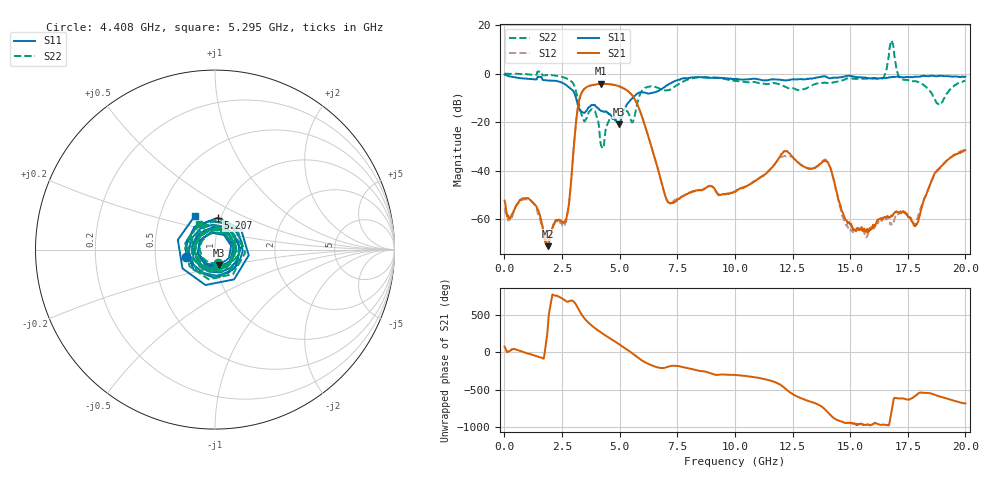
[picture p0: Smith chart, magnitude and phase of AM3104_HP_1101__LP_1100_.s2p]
!Created with skrf (http://scikit-rf.org).
# Hz S RI R 50.0
!freq ReS11 ImS11 ReS21 ImS21 ReS12 ImS12 ReS22 ImS22
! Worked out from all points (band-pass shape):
!   1601 points, 10 MHz to 20 GHz, reference 50 ohm
!   highest |S21| = -4.20 dB at 4.195 GHz (marker M1); lowest = -71.1 dB at 1.872 GHz (marker M2)
!   |S21| within 3 dB of the highest: 3.395 GHz to 5.359 GHz (1.964 GHz wide, 44.9 % of centre)
!   lowest |S11| = -20.9 dB at 4.958 GHz (marker M3), VSWR 1.20, Z = 51.4 - j9.07 ohm
!   |S11| at or under -10 dB: 3.106 GHz to 5.571 GHz (2.465 GHz wide, 56.8 % of centre)
!   |S22| runs from -30.8 to 13.6 dB; largest |S21 - S12| = 0.057
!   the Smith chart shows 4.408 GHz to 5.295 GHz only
!   S11 on the Smith chart (normalised r, x): 4.408 GHz: 0.72, -0.06; 5.207 GHz: 0.97, +0.35; 5.295 GHz: 0.75, +0.30
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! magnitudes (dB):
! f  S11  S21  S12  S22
! 10 MHz  -0.4  -52.3  -55.5  -0.1
! 1.147 GHz  -2.2  -52.3  -52.3  -0.5
! 1.872 GHz  -2.9  -71.1  -67.9  -0.7
! 2.684 GHz  -4.8  -59.9  -60.7  -1.9
! 3.346 GHz  -15.7  -8.0  -8.1  -16.8
! 3.896 GHz  -13.0  -4.6  -4.6  -15.3
! 4.195 GHz  -15.3  -4.2  -4.2  -29.7
! 4.408 GHz  -15.6  -4.3  -4.3  -22.2
! 4.958 GHz  -20.9  -5.2  -5.2  -18.8
! 5.207 GHz  -15.0  -6.3  -6.3  -15.7
! 5.295 GHz  -13.2  -6.8  -6.8  -15.4
! 6.682 GHz  -7.2  -40.0  -40.1  -6.0
! 7.181 GHz  -4.1  -53.3  -53.3  -6.7
! 10.01 GHz  -2.4  -48.7  -48.6  -3.1
! 12.18 GHz  -2.8  -32.0  -34.0  -5.5
! 13.34 GHz  -2.1  -39.2  -39.2  -4.9
! 14.02 GHz  -1.6  -36.4  -36.2  -3.9
! 15.03 GHz  -1.0  -61.9  -64.4  -1.9
! 16.68 GHz  -1.6  -59.2  -60.6  7.2
! 17.86 GHz  -1.4  -62.1  -61.9  -3.2
! 18.83 GHz  -1.0  -39.3  -39.7  -12.6
! 20 GHz  -1.3  -31.6  -31.4  -3.0
